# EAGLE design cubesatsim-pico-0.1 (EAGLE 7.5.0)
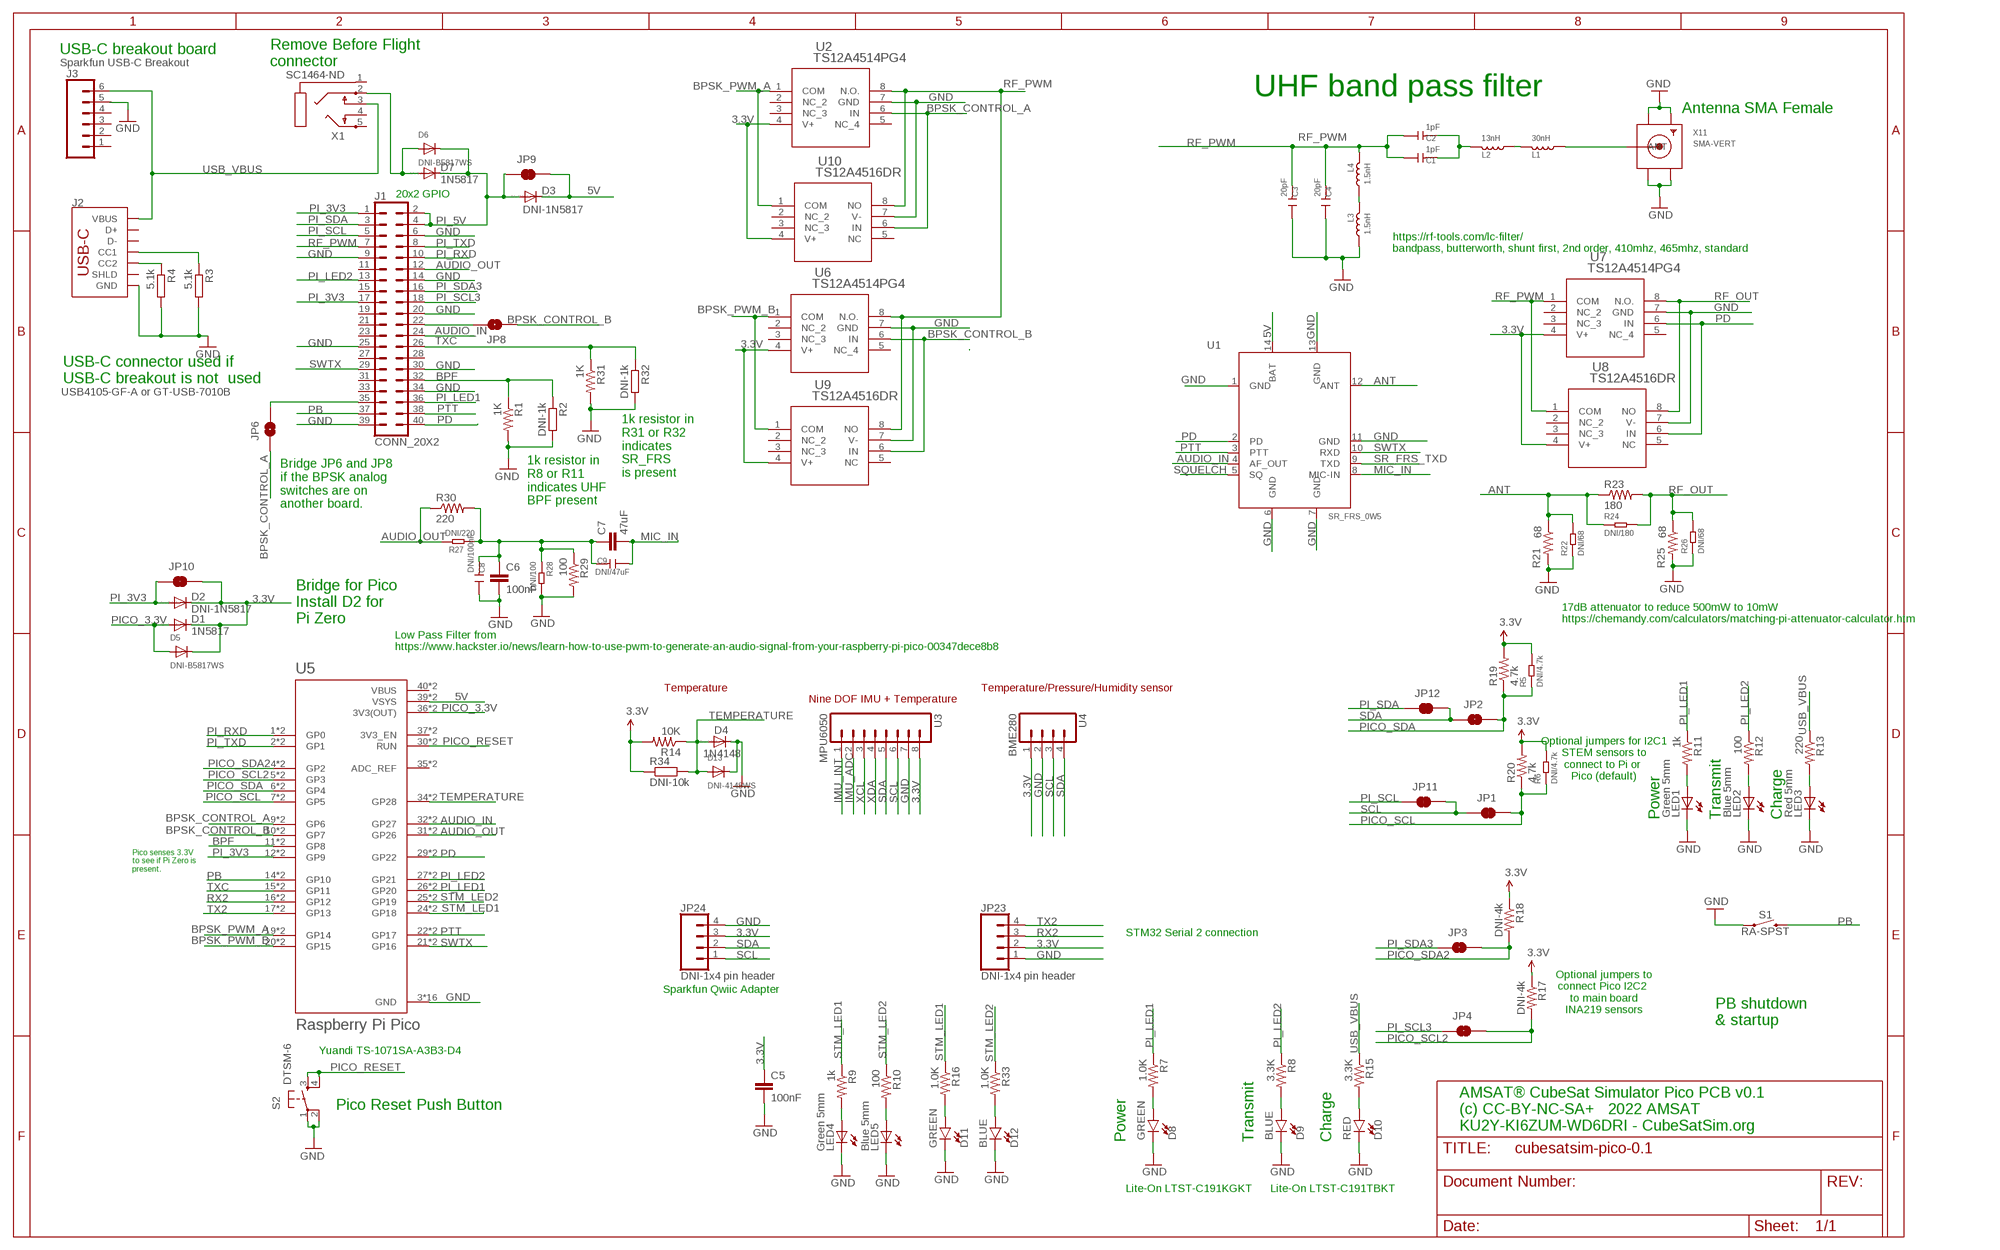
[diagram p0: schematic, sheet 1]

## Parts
C1  1pF  CERAMIC-10PF-50V-5%-NPO(0603)  [C0603]
C2  1pF  CERAMIC-10PF-50V-5%-NPO(0603)  [C0603]
C3  20pF  CERAMIC-10PF-50V-5%-NPO(0603)  [C0603]
C4  20pF  CERAMIC-10PF-50V-5%-NPO(0603)  [C0603]
C5  100nF  CAPPTH  [CAP-PTH-SMALL]
C6  100nF  CAPPTH  [CAP-PTH-SMALL]
C7  47uF  CAPPTH  [CAP-PTH-SMALL]
C8  DNI/100nF  CERAMIC-10PF-50V-5%-NPO(0603)  [C0603]
C9  DNI/47uF  CERAMIC-10PF-50V-5%-NPO(0603)  [C0603]
D1  1N5817  DIODE-D-2.5  [D-2.5]
D2  DNI-1N5817  DIODE-D-2.5  [D-2.5]
D3  DNI-1N5817  DIODE-D-2.5  [D-2.5]
D4  1N4148  DIODE-D-2.5  [D-2.5]
D5  DNI-B5817WS  DIODESOD-323F  [SOD-323F]
D6  DNI-B5817WS  DIODESOD-323F  [SOD-323F]
D7  1N5817  DIODE-D-2.5  [D-2.5]
D8  GREEN  LED-GREEN0603  [LED-0603]
D9  BLUE  LED-BLUE0603  [LED-0603]
D10  RED  LED-BLUE0603  [LED-0603]
D11  GREEN  LED-GREEN0603  [LED-0603]
D12  BLUE  LED-GREEN0603  [LED-0603]
D13  DNI-4148WS  DIODESOD-323F  [SOD-323F]
J1  CONN_20X2  [2X20]
J2  USB4105-GF-A or GT-USB-7010B  USB_C_2-LAYER_PADS  [USB-C-16P-2LAYER-PADS]
J3  Sparkfun USB-C Breakout  CONN_06NO_SILK_FEMALE_PTH  [1X06_NO_SILK]
JP1  JUMPER-SMT_2_NC_TRACE_SILK  [SMT-JUMPER_2_NC_TRACE_SILK]
JP2  JUMPER-SMT_2_NC_TRACE_SILK  [SMT-JUMPER_2_NC_TRACE_SILK]
JP3  JUMPER-SMT_2_NC_TRACE_SILK  [SMT-JUMPER_2_NC_TRACE_SILK]
JP4  JUMPER-SMT_2_NC_TRACE_SILK  [SMT-JUMPER_2_NC_TRACE_SILK]
JP6  JUMPER-SMT_2_NO_SILK  [SMT-JUMPER_2_NO_SILK]
JP8  JUMPER-SMT_2_NO_SILK  [SMT-JUMPER_2_NO_SILK]
JP9  JUMPER-SMT_2_NC_TRACE_SILK  [SMT-JUMPER_2_NC_TRACE_SILK]
JP10  JUMPER-SMT_2_NC_TRACE_SILK  [SMT-JUMPER_2_NC_TRACE_SILK]
JP11  JUMPER-SMT_2_NC_TRACE_SILK  [SMT-JUMPER_2_NC_TRACE_SILK]
JP12  JUMPER-SMT_2_NC_TRACE_SILK  [SMT-JUMPER_2_NC_TRACE_SILK]
JP23  DNI-1x4 pin header  CONN_041X04_NO_SILK  [1X04_NO_SILK]
JP24  DNI-1x4 pin header  CONN_041X04_NO_SILK  [1X04_NO_SILK]
L1  30nH  SMD-FERRITE-CHIP-120-OHM-500MA(0603)  [L0603]
L2  13nH  SMD-FERRITE-CHIP-120-OHM-500MA(0603)  [L0603]
L3  1.5nH  SMD-FERRITE-CHIP-120-OHM-500MA(0603)  [L0603]
L4  1.5nH  SMD-FERRITE-CHIP-120-OHM-500MA(0603)  [L0603]
LED1  Green 5mm  LED3MM  [LED3MM]
LED2  Blue 5mm  LED3MM  [LED3MM]
LED3  Red 5mm  LED3MM  [LED3MM]
LED4  Green 5mm  LED3MM  [LED3MM]
LED5  Blue 5mm  LED3MM  [LED3MM]
R1  1K  RESISTORPTH-1/4W-VERT-KIT  [AXIAL-0.1EZ]
R2  DNI-1k  R-EU_R0603  [R0603]
R3  5.1k  R-EU_R0603  [R0603]
R4  5.1k  R-EU_R0603  [R0603]
R5  DNI/4.7k  SMD-RES-1.2K-1%-1/10W(0603)  [R0603]
R6  DNI/4.7k  SMD-RES-1.2K-1%-1/10W(0603)  [R0603]
R7  1.0K  RESISTOR0603  [0603-RES]
R8  3.3K  RESISTOR0603-RES  [0603-RES]
R9  1k  RESISTORPTH-1/4W-VERT  [AXIAL-0.1]
R10  100  RESISTORPTH-1/4W-VERT  [AXIAL-0.1]
R11  1k  RESISTORPTH-1/4W-VERT-KIT  [AXIAL-0.1EZ]
R12  100  RESISTORPTH-1/4W-VERT-KIT  [AXIAL-0.1EZ]
R13  220  RESISTORPTH-1/4W-VERT-KIT  [AXIAL-0.1EZ]
R14  10K  RESISTORPTH-1/4W-VERT  [AXIAL-0.1]
R15  3.3K  RESISTOR0603-RES  [0603-RES]
R16  1.0K  RESISTOR0603  [0603-RES]
R17  DNI-4k  RESISTORPTH-1/4W-VERT  [AXIAL-0.1]
R18  DNI-4k  RESISTORPTH-1/4W-VERT  [AXIAL-0.1]
R19  4.7k  RESISTORPTH-1/4W-VERT  [AXIAL-0.1]
R20  4.7k  RESISTORPTH-1/4W-VERT  [AXIAL-0.1]
R21  68  RESISTORPTH-1/4W-VERT-KIT  [AXIAL-0.1EZ]
R22  DNI/68  SMD-RES-1.2K-1%-1/10W(0603)  [R0603]
R23  180  RESISTORPTH-1/4W-VERT-KIT  [AXIAL-0.1EZ]
R24  DNI/180  SMD-RES-1.2K-1%-1/10W(0603)  [R0603]
R25  68  RESISTORPTH-1/4W-VERT-KIT  [AXIAL-0.1EZ]
R26  DNI/68  SMD-RES-1.2K-1%-1/10W(0603)  [R0603]
R27  DNI/220  SMD-RES-1.2K-1%-1/10W(0603)  [R0603]
R28  DNI/100  SMD-RES-1.2K-1%-1/10W(0603)  [R0603]
R29  100  RESISTORPTH-1/4W-VERT-KIT  [AXIAL-0.1EZ]
R30  220  RESISTORPTH-1/4W-VERT-KIT  [AXIAL-0.1EZ]
R31  1K  RESISTORPTH-1/4W-VERT-KIT  [AXIAL-0.1EZ]
R32  DNI-1k  R-EU_R0603  [R0603]
R33  1.0K  RESISTOR0603  [0603-RES]
R34  DNI-10k  R-EU_R0603  [R0603]
S1  RA-SPST  [RA-SPST]
S2  DTSM-6  [DTSM-6]
U1  SR_FRS_0W5  [SR_FRS_0W5]
U2  TS12A4514PG4  TS12A4515PG4  [P8_TEX]
U3  MPU6050  M08NO_SILK_FEMALE_PTH  [1X08_NO_SILK]
U4  BME280  M04NO_SILK_ALL_ROUND  [1X04_NO_SILK_ALL_ROUND]
U5  Raspberry Pi Pico  RASPBERRY_PICO-NO_DEBUG  [PICO-PKG-NO_DEBUG]
U6  TS12A4514PG4  TS12A4515PG4  [P8_TEX]
U7  TS12A4514PG4  TS12A4515PG4  [P8_TEX]
U8  TS12A4516DR  [D8]
U9  TS12A4516DR  [D8]
U10  TS12A4516DR  [D8]
X1  SC1464-ND  PG203J  [PG203J]
X11  SMA-VERT  [SMA-VERT]

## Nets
3.3V: C5.1 D1.C D2.C D5.C JP10.2 JP23.2 JP24.3 R5.2 R6.2 R14.P$2 R17.P$1 R18.P$1 R19.P$2 R20.P$2 R34.1 U2.4(V+) U3.8 U4.1 U6.4(V+) U7.4(V+) U8.4(V+) U9.4(V+) U10.4(V+)
5V: D3.C JP9.2 U1.14(BAT) U5.39(VSYS) U5.P$39(VSYS)
ANT: R21.P$1 R22.2 R23.P$1 R24.1 U1.12(ANT)
AUDIO_IN: J1.24 U1.4(AF_OUT) U5.32(GP27) U5.P$32(GP27)
AUDIO_OUT: J1.12 R27.2 R30.P$1 U5.31(GP26) U5.P$31(GP26)
BPF: J1.32 R1.P$1 R2.1 U5.11(GP8) U5.P$11(GP8)
BPSK_CONTROL_A: JP6.1 U2.6(IN) U5.9(GP6) U5.P$9(GP6) U10.6(IN)
BPSK_CONTROL_B: JP8.1 U5.10(GP7) U5.P$10(GP7) U6.6(IN) U9.6(IN)
BPSK_PWM_A: U2.1(COM) U5.19(GP14) U5.P$19(GP14) U10.1(COM)
BPSK_PWM_B: U5.20(GP15) U5.P$20(GP15) U6.1(COM) U9.1(COM)
GND: C3.1 C4.1 C5.2 C6.2 C8.1 D4.C D8.C D9.C D10.C D11.C D12.C D13.C J1.6 J1.9 J1.14 J1.20 J1.25 J1.30 J1.34 J1.39 J2.GND J2.GND2(GND) J3.5 JP23.1 JP24.4 L3.2 LED1.K(C) LED2.K(C) LED3.K(C) LED4.K(C) LED5.K(C) R1.P$2 R2.2 R3.2 R4.2 R21.P$2 R22.1 R25.P$2 R26.1 R28.2 R29.P$2 R31.P$2 R32.2 S1.1 S2.1 S2.2 U1.1(GND) U1.6(GND) U1.7(GND) U1.11(GND) U1.13(GND) U2.7(GND) U3.7 U4.2 U5.3(GND) U5.8(GND) U5.13(GND) U5.18(GND) U5.23(GND) U5.28(GND) U5.33(GND) U5.38(GND) U5.P$3(GND) U5.P$8(GND) U5.P$13(GND) U5.P$18(GND) U5.P$23(GND) U5.P$28(GND) U5.P$33(GND) U5.P$38(GND) U6.7(GND) U7.7(GND) U8.7(V-) U9.7(V-) U10.7(V-) X11.GND1 X11.GND2 X11.GND3 X11.GND4
IMU_ADC: U3.2
IMU_INT: U3.1
MIC_IN: C7.2 C9.1 U1.8(MIC-IN)
N$3: LED4.A R9.P$2
N$4: LED5.A R10.P$2
N$5: C6.1 C7.1 C8.2 C9.2 R27.1 R28.1 R29.P$1 R30.P$2
N$6: LED1.A R11.P$2
N$8: L1.2 X11.ANTENNA(ANT)
N$9: LED2.A R12.P$2
N$10: C1.2 C2.2 L2.1
N$11: LED3.A R13.P$2
N$22: J1.35 JP6.2
N$23: J2.B5(CC2) R4.1
N$24: J2.A5(CC1) R3.1
N$25: J1.22 JP8.2
N$27: D8.A R7.2
N$28: L3.1 L4.2
N$29: D9.A R8.2
N$30: D10.A R15.2
N$31: D11.A R16.2
N$32: D12.A R33.2
N$50: L1.1 L2.2
PB: J1.37 S1.2 U5.14(GP10) U5.P$14(GP10)
PD: J1.40 U1.2(PD) U5.29(GP22) U5.P$29(GP22) U7.6(IN) U8.6(IN)
PI_3V3: D2.A J1.1 J1.17 JP10.1 U5.12(GP9) U5.P$12(GP9)
PI_5V: D3.A D6.C D7.C J1.2 J1.4 JP9.1
PI_LED1: J1.36 R7.1 R11.P$1 U5.26(GP20) U5.P$26(GP20)
PI_LED2: J1.13 R8.1 R12.P$1 U5.27(GP21) U5.P$27(GP21)
PI_RXD: J1.10 U5.1(GP0) U5.P$1(GP0)
PI_SCL: J1.5 JP11.1
PI_SCL3: J1.18 JP4.1
PI_SDA: J1.3 JP12.1
PI_SDA3: J1.16 JP3.1
PI_TXD: J1.8 U5.2(GP1) U5.P$2(GP1)
PICO_3.3V: D1.A D5.A U5.36(3V3(OUT)) U5.P$36(3V3(OUT))
PICO_3.3V1: D6.A D7.A X1.2
PICO_RESET: S2.3 S2.4 U5.30(RUN) U5.P$30(RUN)
PICO_SCL: JP1.2 R6.1 R20.P$1 U5.7(GP5) U5.P$7(GP5)
PICO_SCL2: JP4.2 R17.P$2 U5.5(GP3) U5.P$5(GP3)
PICO_SDA: JP2.2 R5.1 R19.P$1 U5.6(GP4) U5.P$6(GP4)
PICO_SDA2: JP3.2 R18.P$2 U5.4(GP2) U5.P$4(GP2)
PTT: J1.38 U1.3(PTT) U5.22(GP17) U5.P$22(GP17)
RF_OUT: R23.P$2 R24.2 R25.P$1 R26.2 U7.8(N.O.) U8.8(NO)
RF_PWM: C1.1 C2.1 C3.2 C4.2 J1.7 L4.1 U2.8(N.O.) U6.8(N.O.) U7.1(COM) U8.1(COM) U9.8(NO) U10.8(NO)
RX2: JP23.3 U5.16(GP12) U5.P$16(GP12)
SCL: JP1.1 JP11.2 JP24.1 U3.6 U4.3
SDA: JP2.1 JP12.2 JP24.2 U3.5 U4.4
SQUELCH: U1.5(SQ)
SR_FRS_TXD: U1.9(TXD)
STM_LED1: R9.P$1 R16.1 U5.24(GP18) U5.P$24(GP18)
STM_LED2: R10.P$1 R33.1 U5.25(GP19) U5.P$25(GP19)
SWTX: J1.29 U1.10(RXD) U5.21(GP16) U5.P$21(GP16)
TEMPERATURE: D4.A D13.A R14.P$1 R34.2 U5.34(GP28) U5.P$34(GP28)
TX2: JP23.4 U5.17(GP13) U5.P$17(GP13)
TXC: J1.26 R31.P$1 R32.1 U5.15(GP11) U5.P$15(GP11)
USB_VBUS: J2.VBUS1(VBUS) J2.VBUS2(VBUS) J3.6 R13.P$1 R15.1 X1.3
XCL: U3.3
XDA: U3.4
Unconnected: J1.11 J1.15 J1.19 J1.21 J1.23 J1.27 J1.28 J1.31 J1.33 J2.A6(D+) J2.A7(D-) J2.B6(D+) J2.B7(D-) J2.SHLD1(SHLD) J2.SHLD2(SHLD) J2.SHLD3(SHLD) J2.SHLD4(SHLD) J3.1 J3.2 J3.3 J3.4 U2.2(NC_2) U2.3(NC_3) U2.5(NC_4) U5.35(ADC_REF) U5.37(3V3_EN) U5.P$35(ADC_REF) U5.P$37(3V3_EN) U6.2(NC_2) U6.3(NC_3) U6.5(NC_4) U7.2(NC_2) U7.3(NC_3) U7.5(NC_4) U8.2(NC_2) U8.3(NC_3) U8.5(NC) U9.2(NC_2) U9.3(NC_3) U9.5(NC) U10.2(NC_2) U10.3(NC_3) U10.5(NC) X1.1 X1.4 X1.5

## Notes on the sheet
- USB-C breakout board
- Remove Before Flight
  connector
- UHF band pass filter
- Antenna SMA Female
- 20x2 GPIO
- https://rf-tools.com/lc-filter/
  bandpass, butterworth, shunt first, 2nd order, 410mhz, 465mhz, standard
- USB-C connector used if 
  USB-C breakout is not  used
- 1k resistor in 
  R31 or R32
  indicates 
  SR_FRS 
  is present
- 1k resistor in 
  R8 or R11
  indicates UHF 
  BPF present
- Bridge JP6 and JP8
  if the BPSK analog
  switches are on
  another board.
- 17dB attenuator to reduce 500mW to 10mW
  https://chemandy.com/calculators/matching-pi-attenuator-calculator.htm
- Bridge for Pico
  Install D2 for
  Pi Zero
- Low Pass Filter from
  https://www.hackster.io/news/learn-how-to-use-pwm-to-generate-an-audio-signal-from-your-raspberry-pi-pico-00347dece8b8
- Temperature | Temperature/Pressure/Humidity sensor
- Nine DOF IMU + Temperature
- Optional jumpers for I2C1
  STEM sensors to
  connect to Pi or 
  Pico (default)
- Power | Transmit | Charge
- Pico senses 3.3V 
  to see if Pi Zero is
  present.
- STM32 Serial 2 connection
- Optional jumpers to
  connect Pico I2C2 
  to main board
  INA219 sensors
- Sparkfun Qwiic Adapter
- PB shutdown
  & startup
- Yuandi TS-1071SA-A3B3-D4
- Pico Reset Push Button
- AMSAT® CubeSat Simulator Pico PCB v0.1
  (c) CC-BY-NC-SA+   2022 AMSAT
  KU2Y-KI6ZUM-WD6DRI - CubeSatSim.org
- Power | Transmit | Charge
- Lite-On LTST-C191KGKT | Lite-On LTST-C191TBKT

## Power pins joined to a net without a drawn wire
VBUS: U5.40(VBUS) U5.P$40(VBUS)

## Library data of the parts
C1-C4 C8 C9 = Seeed-OPL-Capacitor:CERAMIC-10PF-50V-5%-NPO(0603): 302010097; VALUE: 10pf
C5-C7 = SparkFun-Capacitors:CAP: Capacitor
D1-D4 D7 = diode:DIODE-: DIODE
D5 D6 D13 = adafruit:DIODE: Diode
D8 D11 = SparkFun-LED:LED-GREEN: Green SMD LED; PROD_ID: DIO-00821
D9 = SparkFun-LED:LED-BLUE: Blue SMD LED; PROD_ID: DIO-08575
D10 = SparkFun-LED:LED-BLUE: Blue SMD LED; PROD_ID: DIO-08575; VALUE: BLUE
D12 = SparkFun-LED:LED-GREEN: Green SMD LED; PROD_ID: DIO-00821; VALUE: GREEN
J1 = SparkFun-Connectors-AJ2:CONN_20X2: Multi connection point. Often used as Generic Header-pin footprint for 0.1 inch spaced/style header connections On any of the 0.1 inch spaced packages, you can populate with these: Break Away Headers - Straight (PRT-00116) Break Away Male Headers - Right Angle (PRT-00553) Female Headers (PRT-00115)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
J2 = SparkFun-Connectors:USB_C: USB Type C 16Pin Connector Super Speed pins not available on the 16-pin purely SMD connector so this part is best for USB 2.0 implementations. D1 and D2 are tied together enabling D+/- no matter which way the cable is plugged into the connector. The two channel configuration pins (CC1/2) are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; PROD_ID: CONN-14122
J3 = SparkFun-Connectors-AJ-3:CONN_06: Multi connection point. Often used as Generic Header-pin footprint for 0.1 inch spaced/style header connections On any of the 0.1 inch spaced packages, you can populate with these: Break Away Headers - Straight (PRT-00116) Break Away Male Headers - Right Angle (PRT-00553) Female Headers (PRT-00115)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; PROD_ID: CONN-08437
JP1-JP4 JP9-JP12 = SparkFun-Jumpers:JUMPER-SMT_2_NC_TRACE: Normally closed trace jumper
JP6 JP8 = SparkFun-Jumpers:JUMPER-SMT_2_NO: Normally open jumper
JP23 JP24 = SparkFun-Connectors:CONN_04: Multi connection point. Often used as Generic Header-pin footprint for 0.1 inch spaced/style header connections On any of the 0.1 inch spaced packages, you can populate with these: Break Away Headers - Straight (PRT-00116) Break Away Male Headers - Right Angle (PRT-00553) Female Headers (PRT-00115)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; PROD_ID: CONN-09696
L1-L4 = Seeed-OPL-Inductor:SMD-FERRITE-CHIP-120-OHM-500MA(0603): 303030001; MPN: BLM18AG121SN1D; VALUE: 120
LED1-LED5 = adafruit:LED: LED
R1 R7-R21 R23 R25 R29-R31 R33 = SparkFun-Resistors:RESISTOR: Resistor
R2-R4 R32 R34 = resistor:R-EU_: RESISTOR, European symbol
R5 R6 R22 R24 R26-R28 = Seeed-OPL-Resistor:SMD-RES-1.2K-1%-1/10W(0603): 301010206; MPN: RC0603FR-071K2L; VALUE: 1.2K
S1 = zumradio:RA-SPST
S2 = switch-tact-aj:DTSM-6
U1 = SR_FRS_0W5:SR_FRS_0W5
U2 U6 U7 = TS12A4514:TS12A4515PG4; COPYRIGHT: Copyright (C) 2022 Ultra Librarian. All rights reserved.; MANUFACTURER_PART_NUMBER: TS12A4515PG4; MFR_NAME: Texas Instruments
U3 = SparkFun-Connectors:M08: Header 8 Standard 8-pin 0.1" header. Use with straight break away headers (SKU : PRT-00116), right angle break away headers (PRT-00553), swiss pins (PRT-00743), machine pins (PRT-00117), and female headers (PRT-00115).; PROD_ID: CONN-08438
U4 = SparkFun-Connectors:M04: Header 4 Standard 4-pin 0.1" header. Use with straight break away headers (SKU : PRT-00116), right angle break away headers (PRT-00553), swiss pins (PRT-00743), machine pins (PRT-00117), and female headers (PRT-00115). Molex polarized connector foot print use with SKU : PRT-08231 with associated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
U5 = RpiPico:RASPBERRY_PICO-NO_DEBUG
U8-U10 = TS12A4514-soic:TS12A4516DR; COPYRIGHT: Copyright (C) 2022 Ultra Librarian. All rights reserved.; DIGI-KEY_PART_NUMBER_1: 296-21911-1-ND; DIGI-KEY_PART_NUMBER_2: 296-21911-2-ND; DIGI-KEY_PART_NUMBER_3: 296-21911-6-ND; DIGI-KEY_PART_NUMBER_4: 2156-TS12A4516DR-ND; MANUFACTURER_PART_NUMBER: TS12A4516DR; MFR_NAME: Texas Instruments
X1 = con-hirschmann:PG203J: MIC/HEADPHONE JACK KS-S stereo microphone/headphone jack PG203JN (Schukat); OC_FARNELL: unknown; OC_NEWARK: unknown
X11 = zum_radio:SMA-VERT

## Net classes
1 RF: clearance 0.381 mm

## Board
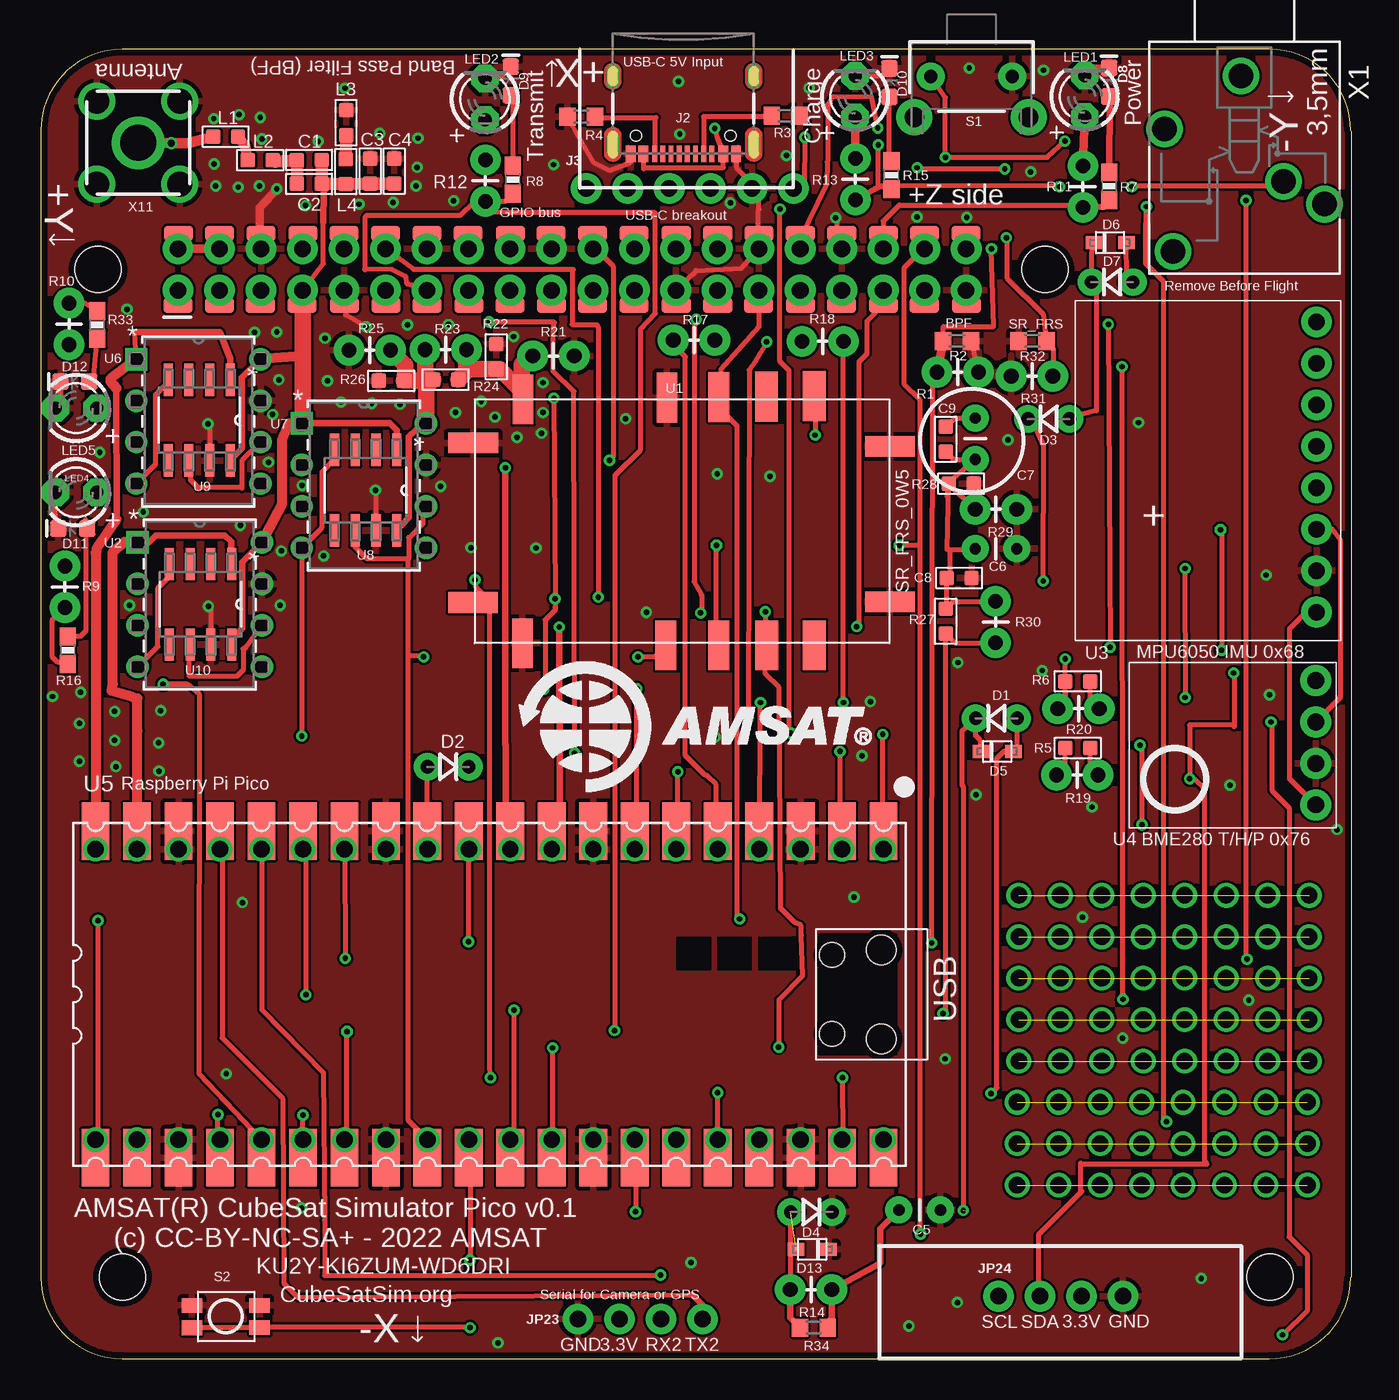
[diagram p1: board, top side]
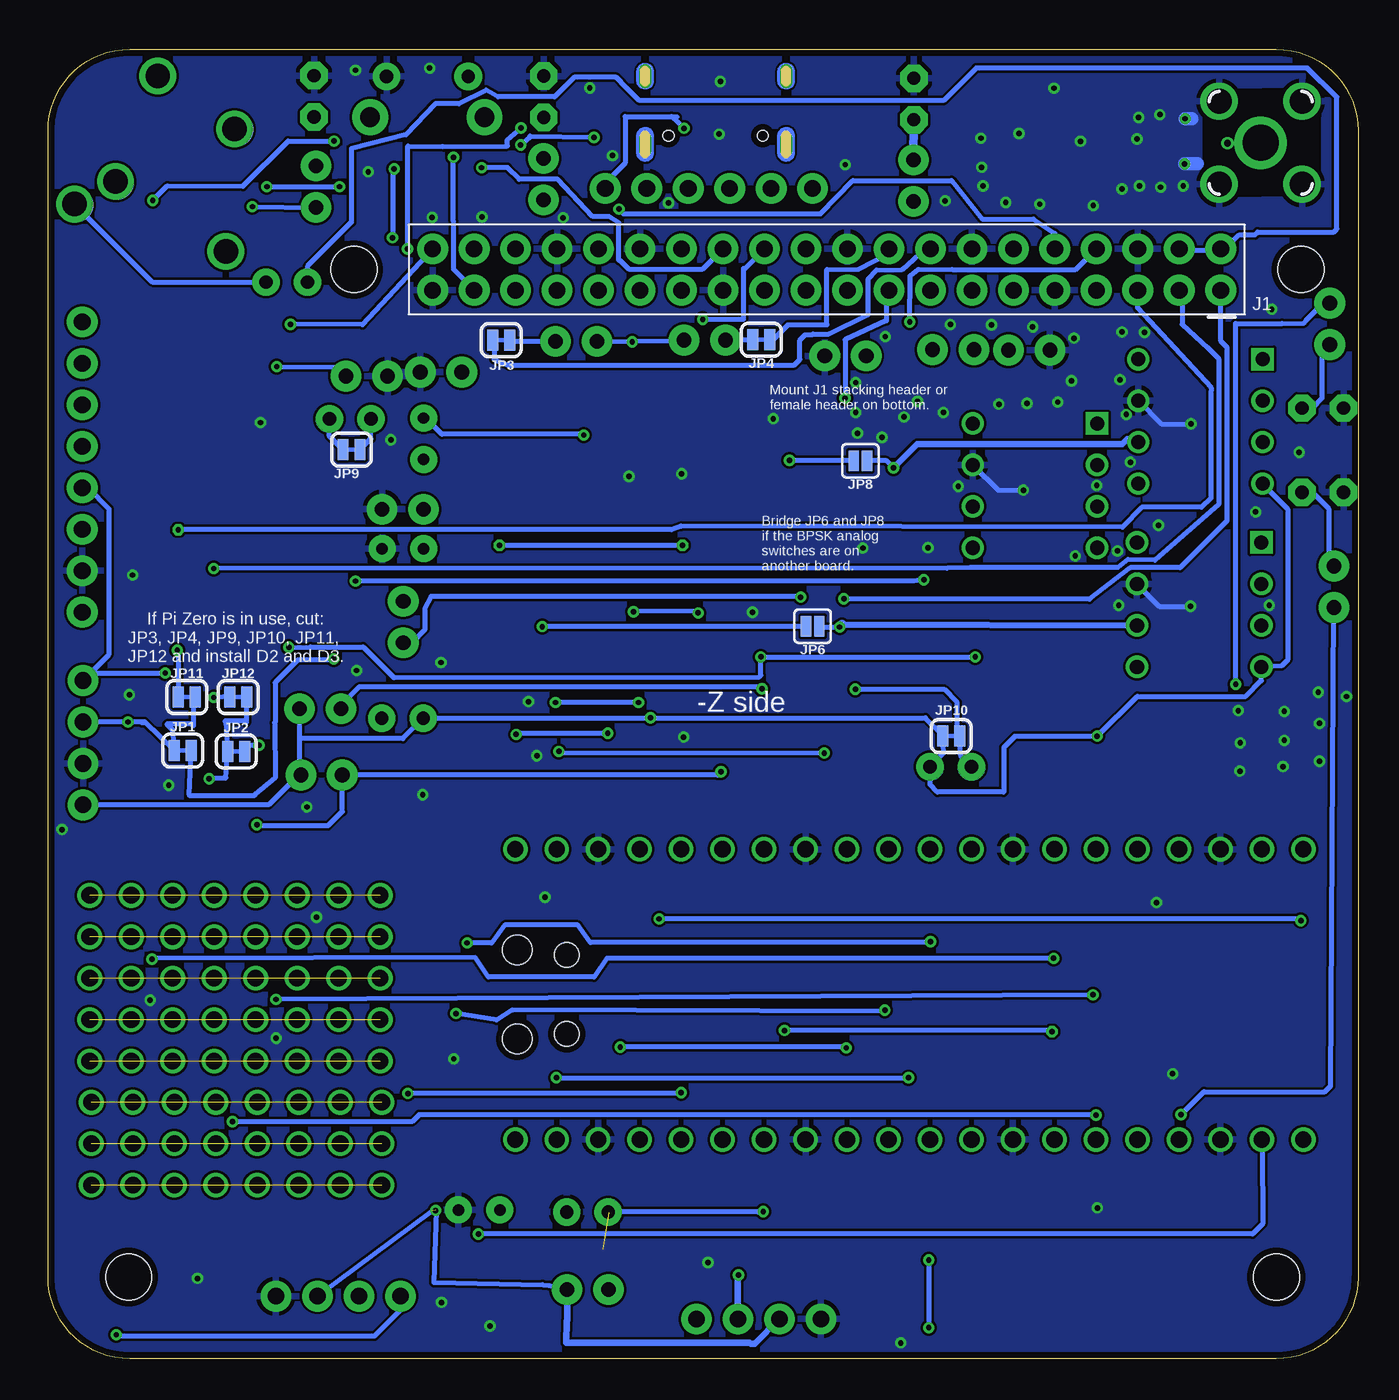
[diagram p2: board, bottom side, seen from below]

Size 80.24 x 80.23 mm. Coordinates in mm from the lower left corner, seen from the top.
Outline: 80.23,5 arc-90 75.23,0 5,0 arc-90 0,5 0,75.23 arc-90 5,80.23 75.23,80.23 arc-90 80.23,75.23
Outline: 80.24,75.2 80.24,4.98
Copper layers (1*16): Top 0.0356mm / dielectric 1.5011mm / Bottom 0.0356mm
Design rules "LaenPCBOrder *": minimum track width 6mil, minimum drill 13mil, track to track 6mil, track to pad 6mil, pad to pad 6mil, via to via 6mil, smd to smd 6mil, copper to edge 15mil, drill to drill 6mil, minimum pad ring 7mil, minimum via ring 7mil, stop-mask expansion 3mil, vias tented up to drill 25mil, thermal gap 10mil
Holes 2.8 mm at 3.5,66.73 61.5,66.73 75.28,5 5,5

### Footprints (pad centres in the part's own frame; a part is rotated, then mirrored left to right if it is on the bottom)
C0603 = smd 0.889 x 0.889: 1 0,0.762; 2 0,-0.762
CAP-PTH-SMALL = drill 0.7 pad 1.651: 1 0,0; 2 2.54,0
D-2.5 = drill 0.813 pad 1.676: A 1.27,0; C -1.27,0 | smd 1.676 x 1.676 bottom: P$1 -1.27,0; P$2 1.27,0
SOD-323F = smd 1 x 0.8: A -1,0; C 1,0
LED-0603 = smd 1 x 1: A -0.877,0; C 0.877,0
2X20 = drill 1.016 pad 1.88: 1 -24.13,-1.27; 2 -24.13,1.27; 3 -21.59,-1.27; 4 -21.59,1.27; 5 -19.05,-1.27; 6 -19.05,1.27; 7 -16.51,-1.27; 8 -16.51,1.27; 9 -13.97,-1.27; 10 -13.97,1.27; 11 -11.43,-1.27; 12 -11.43,1.27; 13 -8.89,-1.27; 14 -8.89,1.27; 15 -6.35,-1.27; 16 -6.35,1.27; 17 -3.81,-1.27; 18 -3.81,1.27; 19 -1.27,-1.27; 20 -1.27,1.27; 21 1.27,-1.27; 22 1.27,1.27; 23 3.81,-1.27; 24 3.81,1.27; 25 6.35,-1.27; 26 6.35,1.27; 27 8.89,-1.27; 28 8.89,1.27; 29 11.43,-1.27; 30 11.43,1.27; 31 13.97,-1.27; 32 13.97,1.27; 33 16.51,-1.27; 34 16.51,1.27; 35 19.05,-1.27; 36 19.05,1.27; 37 21.59,-1.27; 38 21.59,1.27; 39 24.13,-1.27; 40 24.13,1.27 | smd 1.778 x 0.914: P$1 -19.05,2.21; P$4 -16.485,2.21; P$10 -21.59,2.21; P$11 -24.117,2.223; P$12 -13.97,2.21; P$13 -11.43,2.21; P$14 -8.89,2.21; P$16 -6.375,2.21; P$17 -3.785,2.21; P$20 -1.295,2.21; P$21 1.245,2.21; P$22 3.785,2.21; P$23 6.375,2.21; P$27 8.915,2.21; P$28 11.43,2.21; P$29 13.97,2.21; P$30 16.51,2.21; P$31 19.075,2.21; P$32 21.59,2.21; P$33 24.13,2.21; P$41 -19.101,-2.21; P$44 -16.535,-2.21; P$50 -21.59,-2.21; P$51 -24.13,-2.21; P$52 -13.945,-2.21; P$53 -11.405,-2.21; P$54 -8.89,-2.21; P$56 -6.325,-2.21; P$57 -3.81,-2.21; P$60 -1.27,-2.21; P$61 1.245,-2.21; P$62 3.785,-2.21; P$63 6.375,-2.21; P$67 8.915,-2.21; P$68 11.405,-2.21; P$69 13.995,-2.21; P$70 16.485,-2.21; P$71 19.075,-2.21; P$72 21.565,-2.21; P$73 24.155,-2.21
USB-C-16P-2LAYER-PADS = smd 0.3 x 1: A5 -1.25,-0.34; A6 -0.25,-0.34; A7 0.25,-0.34; A8 1.25,-0.34; B5 1.75,-0.34; B6 0.75,-0.34; B7 -0.75,-0.34; B8 -1.75,-0.34 | smd 0.6 x 1: GND -3.225,-0.34; GND2 3.225,-0.34; VBUS1 -2.45,-0.34; VBUS2 2.45,-0.34 | drill 0.4 pad 0.6 long: SHLD1 -4.318,-0.915; SHLD2 4.318,-0.915; SHLD3 -4.318,-5.095; SHLD4 4.318,-5.095 | hole 0.65: -2.89,-1.445; 2.89,-1.445
1X06_NO_SILK = drill 1.016 pad 1.88: 1 0,0; 2 2.54,0; 3 5.08,0; 4 7.62,0; 5 10.16,0; 6 12.7,0 | smd 1.905 x 1.905 bottom: P$2 2.54,0; P$7 0,0; P$8 5.08,0; P$9 7.62,0; P$22 10.16,0; P$23 12.7,0
SMT-JUMPER_2_NC_TRACE_SILK = smd 0.66 x 1.27: 1 -0.521,0; 2 0.521,0
SMT-JUMPER_2_NO_SILK = smd 0.635 x 1.27: 1 -0.406,0; 2 0.406,0
1X04_NO_SILK = drill 1.016 pad 1.88: 1 0,0; 2 2.54,0; 3 5.08,0; 4 7.62,0
L0603 = smd 0.889 x 0.889: 1 -0.762,0; 2 0.762,0
LED3MM = drill 0.813 pad 1.676 octagon: A -1.27,0; K 1.27,0
AXIAL-0.1EZ = drill 0.9 pad 1.88: P$1 0,0; P$2 2.54,0
R0603 = smd 1 x 1.1: 1 -0.85,0; 2 0.85,0
R0603' = smd 0.889 x 0.889: 1 0,0.762; 2 0,-0.762
0603-RES = smd 1.1 x 1: 1 -0.85,0; 2 0.85,0
AXIAL-0.1 = drill 0.9 pad 1.88: P$1 0,0; P$2 2.54,0
RA-SPST = drill 0.8 pad 1.7: 1 -2.5,0; 2 2.5,0 | drill 1.2 pad 2.2: ANCHOR1 -3.5,2.5; ANCHOR2 3.5,2.5
DTSM-6 = smd 1.25 x 0.9: 1 -2.125,0.6; 2 2.025,0.6; 3 -2.125,-0.76; 4 2.025,-0.75
SR_FRS_0W5 = smd 3.048 x 1.27: 1 7.06,-9.694; 2 7.187,-0.926; 3 7.187,2.33; 10 -8.014,2.329; 11 -7.986,-0.846; 12 -7.876,-9.664 | smd 3.048 x 1.397: 4 7.187,5.256; 5 7.187,8.182; 9 -8.042,5.25 | smd 1.27 x 3.048: 6 4.52,12.81; 7 -5.005,12.815; 13 -5.209,-12.717; 14 4.57,-12.722 | smd 3.048 x 1.422: 8 -8.07,8.171
P8_TEX = drill 0.864 pad 1.372 square: 1 0,0 | drill 0.864 pad 1.372: 2 0,-2.54; 3 0,-5.08; 4 0,-7.62; 5 7.62,-7.62; 6 7.62,-5.08; 7 7.62,-2.54; 8 7.62,0
1X08_NO_SILK = drill 1.016 pad 1.88: 1 0,0; 2 2.54,0; 3 5.08,0; 4 7.62,0; 5 10.16,0; 6 12.7,0; 7 15.24,0; 8 17.78,0
1X04_NO_SILK_ALL_ROUND = drill 1.016 pad 1.88: 1 0,0; 2 2.54,0; 3 5.08,0; 4 7.62,0
PICO-PKG-NO_DEBUG = drill 1: 1 -7.62,25.4; 2 -7.62,22.86; 3 -7.62,20.32; 4 -7.62,17.78; 5 -7.62,15.24; 6 -7.62,12.7; 7 -7.62,10.16; 8 -7.62,7.62; 9 -7.62,5.08; 10 -7.62,2.54; 11 -7.62,0; 12 -7.62,-2.54; 13 -7.62,-5.08; 14 -7.62,-7.62; 15 -7.62,-10.16; 16 -7.62,-12.7; 17 -7.62,-15.24; 18 -7.62,-17.78; 19 -7.62,-20.32; 20 -7.62,-22.86; 21 10.16,-22.86; 22 10.16,-20.32; 23 10.16,-17.78; 24 10.16,-15.24; 25 10.16,-12.7; 26 10.16,-10.16; 27 10.16,-7.62; 28 10.16,-5.08; 29 10.16,-2.54; 30 10.16,0; 31 10.16,2.54; 32 10.16,5.08; 33 10.16,7.62; 34 10.16,10.16; 35 10.16,12.7; 36 10.16,15.24; 37 10.16,17.78; 38 10.16,20.32; 39 10.16,22.86; 40 10.16,25.4 | smd 3.5 x 1.7: P$1 -8.73,25.4; P$2 -8.73,22.86; P$3 -8.73,20.32; P$4 -8.73,17.78; P$5 -8.73,15.24; P$6 -8.73,12.7; P$7 -8.73,10.16; P$8 -8.73,7.62; P$9 -8.73,5.08; P$10 -8.73,2.54; P$11 -8.73,0; P$12 -8.73,-2.54; P$13 -8.73,-5.08; P$14 -8.73,-7.62; P$15 -8.73,-10.16; P$16 -8.73,-12.7; P$17 -8.73,-15.24; P$18 -8.73,-17.78; P$19 -8.73,-20.32; P$20 -8.73,-22.86; P$21 11.27,-22.86; P$22 11.27,-20.32; P$23 11.27,-17.78; P$24 11.27,-15.24; P$25 11.27,-12.7; P$26 11.27,-10.16; P$27 11.27,-7.62; P$28 11.27,-5.08; P$29 11.27,-2.54; P$30 11.27,0; P$31 11.27,2.54; P$32 11.27,5.08; P$33 11.27,7.62; P$34 11.27,10.16; P$35 11.27,12.7; P$36 11.27,15.24; P$37 11.27,17.78; P$38 11.27,20.32; P$39 11.27,22.86; P$40 11.27,25.4 | hole 1.8: -1.455,25.27; 3.995,25.27 | hole 1.5: -1.155,22.24; 3.695,22.24
D8 = smd 1.981 x 0.559: 1 -2.464,1.905; 2 -2.464,0.635; 3 -2.464,-0.635; 4 -2.464,-1.905; 5 2.464,-1.905; 6 2.464,-0.635; 7 2.464,0.635; 8 2.464,1.905
PG203J = drill 1.499: 1 -5.004,-0.203; 2 2.845,4.902; 3 1.448,2.388; 4 5.74,-4.369; 5 -1.753,-4.902 | smd 2.159 x 2.159 bottom: P$1 -5.004,-0.178; P$2 -1.727,-5.004; P$3 1.524,2.337; P$4 2.896,4.801; P$5 5.715,-4.369
SMA-VERT = drill 2.2: ANTENNA 0,0 | drill 1.524: GND1 -2.54,2.54; GND2 2.54,2.54; GND3 -2.54,-2.54; GND4 2.54,-2.54

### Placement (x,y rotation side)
C1  16.43,73.44 270 top
C2  16.43,71.98 270 top
C3  20.17,72.75 0 top
C4  21.64,72.75 0 top
C5  52.55,9.11 0 top
C6  57.23,49.62 0 top
C7  57.23,55.09 90 top
C8  56.24,47.82 270 top
C9  55.42,56.33 0 top
D1  58.52,39.24 0 top
D2  24.94,36.26 180 top
D3  61.72,57.57 0 top
D4  47.19,8.98 180 top
D5  58.57,37.2 180 top
D6  65.48,68.37 180 top
D7  65.61,65.96 0 top
D8  65.43,78.2 90 top
D9  28.78,78.28 90 top
D10  51.97,78.17 90 top
D11  1.96,50.87 180 top
D12  2.08,59.86 180 top
D13  47.24,6.7 0 top
J1  32.54,66.73 0 top
J2  39.34,73.48 180 top
J3  33.4,71.7 0 top
JP1  71.98,37.25 0 bottom
JP2  68.71,37.2 0 bottom
JP3  52.48,62.4 0 bottom
JP4  36.55,62.43 180 bottom
JP6  33.4,44.87 180 bottom
JP8  30.48,55.01 180 bottom
JP9  61.65,55.7 0 bottom
JP10  24.92,38.14 180 bottom
JP11  71.73,40.53 0 bottom
JP12  68.58,40.53 0 bottom
JP23  32.89,2.43 0 top
JP24  58.65,3.83 0 top
L1  11.32,74.86 180 top
L2  13.44,73.42 180 top
L3  18.69,75.72 90 top
L4  18.67,72.73 90 top
LED1  63.93,77.34 90 top
LED2  27.2,77.17 90 top
LED3  49.87,77.31 90 top
LED4  2.16,53.08 180 top
LED5  2.16,58.24 180 top
R1  54.89,60.45 0 top
R2  56.11,62.35 0 top
R3  45.62,76.14 0 top
R4  33.1,76.09 180 top
R5  DNI/4.7k  [R0603']  63.5,37.41 90 top
R6  DNI/4.7k  [R0603']  63.5,41.5 90 top
R7  65.43,71.82 90 top
R8  28.91,72.23 90 top
R9  1.47,46.02 90 top
R10  1.73,64.66 270 top
R11  63.82,70.53 90 top
R12  27.23,70.9 90 top
R13  49.89,70.99 90 top
R14  45.9,4.23 0 top
R15  52.1,72.51 90 top
R16  1.65,43.4 90 top
R17  41.27,62.4 180 top
R18  46.61,62.32 0 top
R19  62.2,35.76 0 top
R20  62.28,39.82 0 top
R21  30.12,61.44 0 top
R22  DNI/68  [R0603']  27.89,61.38 0 top
R23  26.06,61.82 180 top
R24  DNI/180  [R0603']  24.79,59.99 270 top
R25  21.41,61.79 180 top
R26  DNI/68  [R0603']  21.46,59.91 90 top
R27  DNI/220  [R0603']  55.42,45.18 0 top
R28  DNI/100  [R0603']  56.36,53.61 90 top
R29  57.23,52.04 0 top
R30  58.47,43.86 90 top
R31  61.98,60.19 180 top
R32  60.73,62.35 180 top
R33  3.45,63.34 270 top
R34  47.35,1.9 180 top
S1  57,78.56 180 top
S2  11.38,2.66 0 top
U1  39.19,50.89 270 top
U2  5.92,50.01 0 top
U3  78.13,63.52 270 top
U4  78.08,33.93 90 top
U5  26.21,23.59 270 top
U6  5.84,61.23 0 top
U7  15.98,57.3 0 top
U8  19.89,53.21 270 top
U9  9.7,57.5 270 top
U10  9.78,46.22 270 top
X1  73.71,73.58 270 top
X11  5.97,74.49 180 bottom

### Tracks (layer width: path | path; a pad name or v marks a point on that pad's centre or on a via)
3.3V  (via drill 0.33)  (1 unrouted)
  Top 0.305: R6.2 64.24,41.29 64.24,40.1 64.52,39.82 R20.P$2 | R19.P$2 64.26,36.24 R5.2 | D5.C 57.56,36.94 57.56,37.86 57.25,38.17 D1.C 56.41,38.45 56.41,35.15 56.49,35.07 v56.49,9.09 | v44.45,62.3 44.48,62.3 43.79,61.13 43.38,60.57 v43.33,39.26 | U4.1 76.48,35.53 76.48,44.72 77.5,45.74 U3.8 | U8.4 17.98,55.09 17.22,54.32 17.22,50.92 U7.4 v15.98,38.14 | U6.4 7.04,54.81 7.04,59.07 7.8,59.84 U9.4 | U2.4 7.16,43.63 7.16,47.21 7.87,47.92 U10.4
  Top 0.406: C5.1 51.41,7.97 51.41,5.86 51.36,5.81 R14.P$2 48.44,2.55 R34.1
  Bottom 0.305: R19.P$2 64.82,35.83 | 64.82,35.83 64.82,37.99 | 64.82,37.99 R20.P$2 | 64.82,37.99 58.5,37.99 D1.C 57.23,39.26 v43.33,39.26 26.49,39.26 25.44,38.21 JP10.2 25.36,37.11 D2.C 26.21,35.17 25.76,34.71 21.72,34.71 21.69,34.74 21.69,37.46 21.01,38.14 v15.98,38.14 13.51,40.58 6.88,40.58 5.92,41.55 U2.4 4.67,42.44 4.32,42.79 4.32,52.06 5.84,53.59 U6.4 | R17.P$1 41.35,62.32 v44.45,62.3 R18.P$1 | 56.49,9.06 v56.49,9.09 56.44,9.09 56.59,4.67 49.94,4.54 49.55,4.49 R14.P$2 | JP24.3 56.69,9.06 | 64.82,35.83 66.73,33.93 U4.1
  Bottom 0.406: JP23.2 36.96,0.91 37.19,0.91 37.26,0.98 48.49,0.98 48.46,2.33 48.44,2.35 R14.P$2
5V  (via drill 0.33)
  Top 0.305: v49.1,17.21 49.15,13.51 U5.39 U5.P$39 | v27.53,17.21 27.48,18.1 27.48,46.42 27.33,46.58 | 27.33,46.58 U1.14 | 27.33,46.58 26.64,47.26 v26.59,47.72 | v61.39,47.64 61.42,55.95 60.71,57.57 D3.C
  Bottom 0.305: v49.1,17.21 v27.53,17.21 | v26.59,47.72 27.2,47.64 v61.39,47.64 | JP9.2 60.45,56.37 D3.C
ANT
  Top 1.016: U1.12 29.44,58.86 29.44,59.28 | R21.P$1 30.1,61.56 29.44,60.9 29.44,59.28 | 29.44,59.28 28.09,60.62 R22.2 26.19,60.62 | R24.1 26.19,60.62 | 26.19,60.62 26.06,60.75 R23.P$1
AUDIO_IN  (via drill 0.33)
  Top 0.305: v31.34,19.04 31.34,13.48 U5.32 U5.P$32 | v45.19,19.09 45.21,19.12 45.21,21.99 46.66,23.44 46.58,25.93 46.56,26.54 46.18,26.71 45.31,27.58 45.21,41.12 44.37,41.95 U1.4 44.37,45.58 v44.37,45.76 | v40.13,63.67 40.03,63.49 40.01,47.59 40.44,46.83 40.46,46.75 40.46,45.81 v40.41,45.69
  Bottom 0.305: v31.34,19.04 31.39,19.09 v45.19,19.09 | J1.24 37.6,66.74 37.64,66.8 37.64,63.67 v40.13,63.67 | v40.41,45.69 40.31,45.79 v44.37,45.76
AUDIO_OUT  (via drill 0.33)
  Top 0.305: v28.98,21.35 28.98,13.66 U5.31 U5.P$31 | v55.24,21.15 55.42,21.33 R27.2 55.98,43.86 R30.P$1 | J1.12 21.65,67.45 21.89,67.45 22.81,66.77 22.84,66.74 32.61,66.74 32.54,66.72 32.54,63.37 32.59,63.34 34.06,63.34 34.14,63.21 v34.14,46.65
  Bottom 0.305: v28.98,21.35 29.06,21.28 51.79,21.35 52.76,20.75 v55.24,21.15 | v34.14,46.65 34.29,46.7 56.77,46.7 57.15,45.97 57.15,44.67 57.96,43.86 R30.P$1
BPF  (via drill 0.33)
  Top 0.305: v26.19,25.55 26.19,31.18 U5.11 U5.P$11 | v54.56,25.47 54.63,61.03 54.61,60.47 R1.P$1 | R2.1 55.27,62.3 55.27,63.24 58.36,63.24 v58.22,67.99 | v51.26,75.41 50.88,77.29 48.51,77.31 | 48.49,77.31 48.51,77.31 | 48.51,77.31 48.18,76.83 48.18,73.35 48.16,73.32 48.13,71.95 46.51,68.63 J1.32
  Top 0.508: R1.P$1 R2.1
  Bottom 0.305: v26.19,25.55 26.39,25.5 47.02,25.5 47.78,26.56 52.25,26.56 53.06,25.47 v54.56,25.47 | v58.22,67.99 58.19,68.04 58.19,74.29 56.06,74.26 52.09,74.29 52.09,74.67 v51.26,75.41
BPSK_CONTROL_A  (via drill 0.33)
  Top 0.305: U2.6 12.52,43.53 12.45,43.53 12.39,43.48 12.39,42.18 12.01,41.8 9.09,41.8 9.09,43.17 9.14,43.22 U10.6 | U5.9 U5.P$9
  Top 0.406: 31.77,33.88 v31.75,44.82
  Top 0.61: U5.9 31.77,33.88
  Bottom 0.305: JP6.1 32.94,44.82 v31.75,44.82
  Bottom 0.406: 31.6,44.98 U2.6
  Bottom 0.61: v31.75,44.82 31.6,44.98
BPSK_CONTROL_B  (via drill 0.33)
  Top 0.305: U6.6 12.32,55.01 12.32,53.33 12.29,53.36 9.63,53.36 9.17,53.82 9.17,54.5 9.07,54.6 U9.6
  Top 0.406: v28.45,54.58 28.45,37.64 28.47,37.64 28.47,33.09 28.75,32.71 U5.P$10 U5.10
  Top 0.61: U5.P$10 28.75,32.09
  Bottom 0.305: v28.45,54.58 28.88,55.01 JP8.1
  Bottom 0.406: v28.45,54.58 27,56.02 14.45,56.02 14.15,56.33 U6.6
BPSK_PWM_A
  Top 0.305: U10.1 11.63,48.81 11.66,48.84 | U5.19 U5.P$19
  Top 0.406: 11.66,48.84 11.66,50.06 11.28,50.44 7.04,50.44 6.6,50.01 U2.1
  Top 0.61: U5.P$19 5.92,38.47 5.92,40.45 5.64,40.53 4.34,40.91 4.42,41.34 4.42,49.45 5.13,50.06 U2.1
BPSK_PWM_B
  Top 0.305: U6.1 5.77,62.88
  Top 0.406: 5.77,62.88 10.97,62.88 11.61,61.28 U9.1 | 4.62,59.45 4.65,51.43
  Top 0.61: U6.1 4.27,60.04 4.27,59.89 4.62,59.45 | 4.65,51.43 3.4,49.62 3.4,49.42 3.35,49.37 U5.P$20 U5.20
GND  (via drill 0.33)
  Top 0.305: J1.9 18.67,63.95 v19.93,63.21 | J1.25 40.13,66.67 42.93,66.82 J1.30 43.94,70.38 43.97,70.4 43.97,71.04 43.56,71.44 J3.5 43.56,72 42.6,72.97 42.6,73.79 J2.GND | v20.5,53.21 20.52,53 U8.7 | v10.24,57.27 10.34,57.17 U9.7 | v10.26,46.09 10.41,45.94 U10.7 | J2.GND2 36.07,73.25 34.85,72.79 33.86,73.27 R4.2 | R2.2 R1.P$2 | D9.C 28.07,78.44 LED2.K | D10.C 51.5,78.58 LED3.K | D11.C 0.89,51.69 LED4.K | LED5.K 1.21,58.55 D12.C | J1.34 48.77,68.28 48.77,69.89 48.74,69.92 48.67,69.92 48.69,69.95 48.77,69.95
  Top 0.406: J1.6 13.41,68 | LED1.K 64.4,79.08 D8.C
  Top 0.508: 13.41,68 13.41,70.53 v14.45,71.66
  Bottom 0.305: U7.7 22.05,53.21 v20.5,53.21 | U6.7 12.04,57.27 v10.24,57.27 | U2.7 12.17,46.09 v10.26,46.09
  Bottom 0.813: 9.84,73.2 v10.62,73.2 | 10.2,75.96 v10.59,75.96
  other vias: 18.62,77.83 16.22,70.64 73.98,21.97 16.99,74.58 22.97,71.85 11.35,17.46 12.09,71.77 67.22,57.35 13.54,74.72 53.16,2 20.76,75.06 21.58,70.83 28,0.97 56.16,42.65 75.04,48.01 64.38,33.8 79.37,32.42 57.28,34.55 66.26,19.64 61.33,42.16 50.8,40.25 6.27,51.87 63.79,27.05 39.81,5.89 12.34,27.95 31.41,73.15 25.4,57.97 26.97,58.66 27.81,57.69 29.16,56.45 30.66,56.7 30.76,57.97 30.76,59.8 24.48,53.45 22.45,63.33 22,58.48 20.27,58.53 18.39,58.6 17.55,59.9 17.4,62.52 14.45,62.9 14.58,59.98 12.22,51.06 14.66,46.16 13.08,62.87 23.05,72.99 23.1,74.77 10.71,71.85 47.05,77.84 19.49,70.73 25.29,70.94 42.23,70.81 44.65,54.06 41.43,54.21 26.34,49.69 17.32,49.18 37.08,45.73 41.3,38.08 50.29,36.94 75.25,40.67 15.96,9.24 72.83,35.13 30.33,49.66 2.36,38.92 60.62,72.71 45.66,73.7 28.96,62.62 24.97,63.35 35.81,57.59 13.94,54.92 16,53.5 71.07,4.92 56.13,3.45 56.86,79.06 61.4,78.94 56.7,69.92 13.38,71.85 13.44,76.04 12.14,76.22 14.2,57.84 14.73,49.49 2.44,40.82 5.43,46.16 2.36,36.61 4.52,39.66 4.52,37.88 4.6,36.28 7.34,39.71 7.24,36 7.21,37.73 0.71,40.57 3.61,55.53 5.28,64.29 48.68,69.89 53.66,69.95 39.13,75.03 39.05,78.25 49.8,28.28 55.38,18.37 59.23,56.29
  pour Bottom: 0,75.23 0,5 arc90 5,0 75.23,0 arc90 80.23,5 80.23,75.23 arc90 75.23,80.23 5,80.23 arc90
  pour Top: 0,75.23 0,5 arc90 5,0 75.23,0 arc90 80.23,5 80.28,75.23 arc90 75.23,80.23 5,80.23 arc90
MIC_IN  (via drill 0.33)
  Top 0.305: U1.8 47.42,58.91 v47.42,56.58 | C9.1 55.96,57.63 C7.2
  Bottom 0.305: v47.42,56.58 47.47,56.63 56.11,56.63 57.1,57.63 C7.2
N$1
  cutout Top: 2.55,77.53 2.58,71.47 9.27,71.44 9.19,77.49
N$2
  cutout Bottom: 2.5,77.62 2.55,71.46 9.31,71.41 9.23,77.56
N$3
  Bottom 0.305: R9.P$2 1.78,48.94 1.78,52.04 2.82,53.08 LED4.A
N$4
  Bottom 0.305: R10.P$2 2.21,61.64 2.21,58.84 2.82,58.23 LED5.A
N$5
  Top 0.305: C9.2 55.91,55.09 C7.1 55.6,53.66 55.58,53.61 R29.P$1 57.28,52.06 55.58,53.54 55.5,52.82 R28.1 55.5,49.57 55.52,49.55 55.7,49.55 | C6.1 57.15,49.55 55.7,49.55 | R30.P$2 55.88,46.4 R27.1 55.47,45.99 C8.2 55.7,48.05 55.7,49.55
N$6
  Top 0.508: LED1.A R11.P$2
N$7  (via drill 1.02)  (7 unrouted)
  other vias: 59.79,15.72 62.33,15.72 64.87,15.72 69.95,15.72 67.41,15.72 72.49,15.72 75.03,15.72 77.57,15.72
N$8  (via drill 0.41)
  Top 0.635: L1.2 9,74.47 v7.99,74.47 X11.ANTENNA
N$9
  Bottom 0.508: LED2.A R12.P$2
N$10
  Top 0.508: L2.1 14.36,73.34 | C1.2 15.73,73.32
  Top 0.762: 14.36,73.34 C1.2 | 15.73,73.32 C2.2
N$11
  Top 0.508: LED3.A R13.P$2
N$12  (via drill 1.02)  (7 unrouted)
  other vias: 59.79,13.18 62.33,13.18 64.87,13.18 69.95,13.18 67.41,13.18 72.49,13.18 75.03,13.18 77.57,13.18
N$14  (via drill 1.02)  (7 unrouted)
  other vias: 59.89,28.39 62.43,28.39 64.97,28.39 70.05,28.39 67.51,28.39 72.59,28.39 75.13,28.39 77.67,28.39
N$15  (via drill 1.02)  (7 unrouted)
  other vias: 59.89,25.85 62.43,25.85 64.97,25.85 70.05,25.85 67.51,25.85 72.59,25.85 75.13,25.85 77.67,25.85
N$16  (via drill 1.02)  (7 unrouted)
  other vias: 59.89,23.31 62.43,23.31 64.97,23.31 70.05,23.31 67.51,23.31 72.59,23.31 75.13,23.31 77.67,23.31
N$17  (via drill 1.02)  (7 unrouted)
  other vias: 59.89,20.77 62.43,20.77 64.97,20.77 70.05,20.77 67.51,20.77 72.59,20.77 75.13,20.77 77.67,20.77
N$18  (via drill 1.02)  (7 unrouted)
  other vias: 59.89,18.23 62.43,18.23 64.97,18.23 70.05,18.23 67.51,18.23 72.59,18.23 75.13,18.23 77.67,18.23
N$19  (via drill 1.02)  (7 unrouted)
  other vias: 59.79,10.64 62.33,10.64 64.87,10.64 69.95,10.64 67.41,10.64 72.49,10.64 75.03,10.64 77.57,10.64
N$20
  Top 0.305: 27.33,70.91 27.3,70.91
N$22  (via drill 0.33)
  Top 0.305: v49.96,44.85 50.11,45 50.11,61.08 50.6,61.56 50.6,63.57 51.59,64.56 J1.35
  Bottom 0.305: JP6.2 33.83,44.85 v49.96,44.85
N$23
  Top 0.305: R4.1 34,76.04 37.67,76.04 37.59,75.97 J2.B5
N$24
  Top 0.305: R3.1 44.72,76.09 40.59,76.09 J2.A5
N$25  (via drill 0.33)
  Top 0.305: v34.82,55.03 35.08,55.29 35.08,66.9 33.98,68 J1.22
  Bottom 0.305: JP8.2 30.91,55.03 v34.82,55.03
N$27
  Top 0.406: D8.A 65.46,77.3 R7.2
N$28
  Top 0.762: L3.1 L4.2
N$29
  Top 0.305: D9.A 28.91,77.27 R8.2
N$30
  Top 0.305: R15.2 51.97,73.49 D10.A
N$31
  Top 0.305: D11.A 2.74,51.41 2.74,44.57 2.42,44.25 R16.2
N$32
  Top 0.305: D12.A 3.25,60.15 R33.2
N$50
  Top 0.635: L1.1 12.51,74.28 L2.2
PB  (via drill 0.33)
  Top 0.305: v18.64,24.53 18.62,31.21 U5.14 U5.P$14 | v73.86,24.48 73.81,24.38 v73.81,70.96 | S1.2 55.4,77.26 v55.4,73.6 61.65,73.6 v62.71,74.59
  Bottom 0.305: J1.37 55.38,66.74 55.38,69.67 55.4,69.68 v55.4,73.6 | v18.64,24.53 46,24.53 46.79,23.39 53.26,23.39 54.08,24.58 73.86,24.53 v73.86,24.48 | v73.81,70.96 72.92,71.85 68.29,71.83 65.53,74.59 v62.71,74.59
PD  (via drill 0.33)
  Top 0.305: U7.6 23.39,52.01 23.39,51.15 22.55,50.31 22.53,50.31 22.53,49.02 22.5,48.99 | 22.5,48.99 19.99,48.99 19.25,49.73 U8.6 | 22.5,43.05 22.5,14.6 U5.29 U5.P$29 | 22.5,43.05 22.5,48.99 | U1.2 37.55,42.99 v36.58,42.99 | v23.44,42.99 23.39,43.05 22.5,43.05 | v65.38,63.37 65.38,63.31 v65.48,43.58
  Bottom 0.305: v23.44,42.99 v36.58,42.99 36.58,41.88 36.65,41.78 59.05,41.72 60.94,43.6 64.16,43.6 v65.48,43.58 | J1.40 60.97,63.34 v65.38,63.37
PI_3V3  (via drill 0.33)
  Top 0.305: U5.12 U5.P$12 D2.A | v31.42,58.84 31.49,46.66 | 31.49,46.66 v31.49,46.55 | v31.49,46.55 31.5,46.04 31.5,45.86 30.89,45.26 30.89,41.12 v30.79,41.01 | v31.49,46.55 31.49,46.66
  Bottom 0.305: D2.A 24.32,36.91 JP10.1 24.56,38.31 24.56,40.23 25.35,41.01 v30.79,41.01 | J1.17 28.88,65.31 28.88,63.59 31.42,62.43 v31.42,58.84 | J1.1 8.43,65.44 8.43,62.38 8.03,61.97 8.03,51.33 10.9,48.46 13.95,48.46 16.46,46.53 v31.49,46.55
PI_5V
  Top 0.305: D6.C 64.34,67.69 D7.C 64.64,65.32 64.64,58.08 62.28,57.47 D3.A
  Top 0.508: J1.2 J1.4
  Bottom 0.305: JP9.1 62.99,56.52 D3.A | J1.4 10.87,67.91 8.2,67.91 7.26,68.85 6.33,68.85 6.15,69.03 1.47,69.03 1.29,69.21 1.29,77.31 1.35,77.31 3.1,79.06 23.39,79.06 25.38,77.08 44.02,77.08 45.11,78.17 45.11,78.2 45.41,78.5 48.01,78.5 49.2,77.31 52.68,77.31 53.39,77.72 55.07,76.88 56.52,76.88 58.32,74.97 61.65,74.14 61.65,69.61 64.34,66.92 D7.C
PI_LED1  (via drill 0.33)
  Top 0.305: v16.05,14.93 U5.26 U5.P$26 | v68.94,14.52 68.78,14.67 68.78,65.98 67.67,67.1 67.67,69.26 v67.72,70.58 | J1.36 51.59,69.69 52.58,70.68 63.72,70.68 R11.P$1
  Top 0.406: R7.1 65.11,70.58 R11.P$1
  Bottom 0.305: v16.05,14.93 16.51,14.95 57.51,14.95 57.94,14.52 v68.94,14.52 | v67.72,70.58 R11.P$1
PI_LED2  (via drill 0.33)
  Top 0.305: 18.75,13.58 v18.75,20.03 | 35.18,20.16 35.18,54.12 36.73,55.67 36.73,63.06 37.64,64.03 37.64,70.17 37.59,70.22 28.65,70.22 27.62,70.25 R12.P$1 | J1.13 22.41,65.86 22.38,66.29 21.51,66.72 19.84,66.74 19.86,66.69 19.86,69.89 19.94,70.05 25.68,70.05 26.53,70.9 R12.P$1 | R8.1 28.42,70.9 R12.P$1 | U5.27 U5.P$27
  Top 0.406: U5.27 18.75,13.58 | v35.13,20.11 35.18,20.16
  Bottom 0.305: 18.82,20.11 v35.13,20.11
  Bottom 0.406: v18.75,20.03 18.82,20.11
PI_RXD  (via drill 0.33)
  Top 0.305: U5.1 51.56,31.26 | 51.56,31.26 v51.56,38.24 | v45.95,38.32 45.82,38.45 45.82,60.55 45.26,61.1 v45.26,70.43 | 51.56,31.26 U5.P$1
  Bottom 0.305: v51.56,38.24 51.49,38.32 v45.95,38.32 | v45.26,70.43 44.98,70.15 32.92,70.15 30.94,72.18 24.89,72.18 23.01,69.82 19.89,69.82 18.57,68.93 J1.10
PI_SCL  (via drill 0.33)
  Top 0.305: v72.25,50.78 72.31,50.72 v72.31,43.4
  Bottom 0.305: J1.5 13.51,65.44 13.51,64.38 8.99,59.48 8.99,59.28 9.02,59.25 9.02,52.7 9.58,52.16 13.23,52.16 14.43,50.95 41.45,51 42.04,50.79 72.24,50.79 v72.25,50.78 | v72.31,43.4 72.25,43.34 JP11.1
PI_SCL3
  Bottom 0.305: J1.18 28.73,67.71 30.58,66.74 32.54,66.72 32.54,63.37 32.51,63.34 34.9,63.34 35.81,62.43 JP4.1 36.11,62.4
PI_SDA  (via drill 0.33)
  Top 0.305: v70.08,48.4 70.05,48.43 v70.08,40.51
  Bottom 0.305: J1.3 10.77,65.28 10.77,63.37 9.17,61.92 8.53,61.28 8.53,52.32 12.42,48.91 14.1,48.96 14.71,48.48 23.72,48.48 25.17,48.43 v70.08,48.4 | v70.08,40.51 69.2,40.59 JP12.1
PI_SDA3
  Bottom 0.305: J1.16 26.51,68 27.91,66.72 29.49,66.69 30,66.14 30,63.95 32.41,62.78 33.38,62.78 33.43,62.73 33.86,62.73 34.19,62.4 34.19,61.21 34.52,60.88 51.94,60.88 51.99,60.83 52.91,61.21 52.91,62.31 JP3.1
PI_TXD  (via drill 0.33)
  Top 0.305: U5.2 48.95,31.34 | 48.95,31.34 v48.95,37.2 | v32.69,37.1 32.64,59.25 31.39,60.47 31.39,63.04 31.45,63.49 v27.46,63.52 | 48.95,31.34 U5.P$2
  Bottom 0.305: v48.95,37.2 48.87,37.13 v32.69,37.1 | v27.46,63.52 27.43,66.34 26.92,66.74 24.87,66.72 17.3,66.72 16.03,67.99 J1.8
PICO_3.3V  (via drill 0.33)
  Top 0.305: D1.A 59.79,36.99 D5.A 58.98,37.2 58.55,36.77 58.55,16.61 v58.19,16.25 | v41.45,16.3 U5.36 U5.P$36
  Bottom 0.305: v58.19,16.25 41.5,16.25 v41.45,16.3
PICO_3.3V1
  Top 0.305: D7.A 66.51,66.33 D6.A
  Bottom 0.305: X1.2 73.84,65.96 D7.A
PICO_RESET  (via drill 0.33)
  Top 0.305: S2.3 S2.4 26,1.91 v26.29,1.9 | v26.29,6.04 26.29,13.35 U5.P$30
  Top 0.406: U5.30 26.29,13.35
  Bottom 0.305: v26.29,6.04 v26.29,1.9
PICO_SCL  (via drill 0.33)
  Top 0.305: U5.7 36.5,31.34 | 36.5,31.34 v36.5,41.04 | R20.P$1 62.76,40.3 | 62.76,40.3 R6.1 | 62.76,40.3 62.74,40.33 v62.74,42.87 | 36.5,31.34 U5.P$7
  Bottom 0.305: v36.5,41.04 36.6,41.14 61.19,41.14 62.28,40.05 R20.P$1 | v62.74,42.87 62.79,42.82 64.92,42.82 66.32,41.42 66.32,38.98 66.34,38.96 66.32,35.58 67.53,34.57 67.61,34.49 71.53,34.49 71.56,34.52 JP1.2
PICO_SCL2
  Top 0.305: U5.5 41.35,31.31 | 41.35,31.31 41.35,35.17 40.79,35.73 40.69,35.73 39.47,36.95 39.47,61.38 38.73,62.12 R17.P$2 | 41.35,31.31 U5.P$5
  Bottom 0.305: 38.58,62.25 R17.P$2 37.1,62.4 JP4.2
PICO_SDA  (via drill 0.33)
  Top 0.305: U5.6 39.01,31.31 | 39.01,31.31 v39.01,35.96 | R19.P$1 62.74,36.29 R5.1 | v67.31,37.59 67.44,37.46 v67.44,32.71 | 39.01,31.31 U5.P$6
  Bottom 0.305: v39.01,35.96 39.22,35.76 R19.P$1 62.2,33.52 63.07,32.66 67.39,32.66 v67.44,32.71 | JP2.2 68.24,37.59 v67.31,37.59
PICO_SDA2  (via drill 0.33)
  Top 0.305: U5.4 44.04,31.26 | 44.04,31.26 v44.07,40.2 | v49.15,40.2 R18.P$2 | 44.04,31.26 U5.P$4
  Bottom 0.305: 49.2,62.38 R18.P$2 51.88,62.32 JP3.2 | v44.07,40.2 v49.15,40.2
PTT  (via drill 0.33)
  Top 0.305: v53.87,7.64 53.85,7.66 53.85,49.85 | 53.85,49.85 53.85,58.72 52.88,59.68 52.88,66.85 54.03,68 J1.38 | U1.3 41.38,43.78 v41.38,49.83 | v52.58,49.83 52.6,49.85 53.85,49.85 | U5.P$22 U5.22
  Bottom 0.305: v53.87,7.64 6.45,7.64 5.84,8.25 5.87,12.9 U5.22 | v41.38,49.83 v52.58,49.83
RF_OUT
  Top 0.406: U8.8 22.53,51.53 22.53,56.48 23.39,57.29 U7.8
  Top 1.016: 23.55,59.91 23.95,59.91 R24.2 23.6,59.56 U7.8 | 23.55,59.91 R26.2 22.33,60.01 22.33,60.88 R25.P$1 | R23.P$2 23.55,61.79 23.55,59.91
RF_PWM
  Top 0.305: J1.7 17.3,67.09 17.31,69.61 | 11.68,44.06 U10.8 | 11.61,55.06 U9.8
  Top 0.406: 17.31,69.61 17.34,71.52 17.79,71.97 | U7.1 16,57.32 21.36,57.32 21.79,56.89 U8.1 | 11.68,44.06 12.34,44.72 12.34,48.81 U2.8 | U6.8 12.32,60.09 12.32,55.77 11.61,55.06
  Top 0.508: 17.79,71.97 C2.1
  Top 0.61: U6.8 15.98,61.41 16.03,61.46 16.03,57.35 U7.1 15.19,57.29 14.78,56.3 14.78,52.37 U2.8
  Top 0.762: C4.2 C3.2 L4.1 17.79,71.97 | C2.1 C1.1
  Top 1.016: U7.1 16.03,57.35 J1.7
RX2  (via drill 0.33)
  Top 0.305: 13.54,31.21 13.54,21.35 17.3,17.52 17.37,8.45 17.37,5.1 v37.95,5.12 | U5.16 U5.P$16
  Top 0.406: U5.16 13.54,31.21
  Bottom 0.406: v37.95,5.12 37.97,5.12 JP23.3
SCL  (via drill 0.33)
  Top 0.305: U4.3 79.6,40.53 79.58,40.58 79.6,40.63 79.6,50.16 79.1,50.82 U3.6 | v75.34,39.01 75.39,38.96 75.39,34.82 76.45,33.75 76.45,7.46 77.55,6.37 77.55,2.91 76.1,1.47 v76.05,1.47
  Bottom 0.305: JP11.2 71.32,40.29 71.32,38.78 71.42,38.88 72.95,38.88 72.61,38.54 JP1.1 | JP1.1 74.31,39.01 74.52,39.01 | U4.3 v75.34,39.01 74.52,39.01 | JP1.1 74.26,38.96 74.47,38.96 74.52,39.01 | v76.05,1.47 75.97,1.39 60.22,1.39 58.65,2.97 JP24.1
SDA  (via drill 0.33)
  Top 0.305: v73.05,42 73.08,41.98 73.08,38.7 72.95,38.83 70.38,38.83 70.36,38.8 v70.36,35.53 70.64,35.53 71.27,34.89 71.27,12.08 71.42,11.93 63.73,11.93 63.68,11.98 63.68,10.2 63.75,10.25 61.11,7.61 61.11,3.91 JP24.2
  Bottom 0.305: U4.4 77.62,42 | 77.62,42 v73.05,42 | v70.36,35.53 70.31,35.58 69.32,35.58 69.33,35.59 JP2.1 69.33,38.99 69.39,39.06 68.2,39.06 68.1,38.96 68.1,40.49 JP12.2 | 77.62,42 76.48,43.15 76.48,52.06 77.78,53.36 U3.5
STM_LED1  (via drill 0.33)
  Top 0.305: v10.85,14.95 10.85,13.56 U5.24 U5.P$24 | R16.1 1.54,42.66 1.04,42.66 0.71,42.99 0.71,45.26 R9.P$1 1.65,46.2
  Bottom 0.305: v10.85,14.95 9.45,16.35 2.03,16.35 1.68,16.71 R9.P$1
STM_LED2  (via drill 0.33)
  Top 0.305: v7.49,41.32 8.97,41.32 9.73,40.68 9.7,17.44 U5.25 U5.P$25 | R33.1 2.68,64.66 R10.P$1
  Bottom 0.305: v7.49,41.32 7.49,63.42 4.65,63.42 3.3,63.44 3.17,63.62 2.13,64.66 R10.P$1
SWTX  (via drill 0.33)
  Top 0.305: v3.5,26.84 3.5,13.58 U5.21 U5.P$21 | v42.8,26.94 42.65,27.1 42.65,57.14 41.71,58.08 41.71,58.41 41.52,58.6 U1.10 41.63,59.02 41.66,60.62 43.99,63.22 J1.29
  Bottom 0.305: v3.5,26.84 3.61,26.94 v42.8,26.94
TEMPERATURE  (via drill 0.33)  (1 unrouted)
  Top 0.305: U5.34 36.42,13.38 | 36.42,13.38 v36.42,9.01 | D4.A 45.9,8.96 R14.P$1 | 36.42,13.38 U5.P$34
  Top 0.406: R34.2 45.9,2.5 R14.P$1
  Bottom 0.305: v36.42,9.01 36.75,8.98 D4.A
TX2
  Top 0.305: 11.1,31.08 11.1,19.65 14.81,15.94 14.88,4.62 15.75,3.75 39.9,3.91 | U5.17 U5.P$17
  Top 0.406: U5.17 11.1,31.08 | 39.9,3.91 40.51,3.29 JP23.4
TXC  (via drill 0.33)
  Top 0.305: 16.23,31.21 v16.23,22.29 | 66.27,22.29 v66.22,60.77 | v53.67,72.97 53.75,72.89 v59.03,72.89 | v59.13,68.68 59.16,68.65 59.16,66.21 61.38,63.99 R32.1 62,61.9 R31.P$1 | U5.15 U5.P$15
  Top 0.406: U5.15 16.23,31.21 | v66.27,22.02 66.27,22.29
  Bottom 0.305: v16.23,22.29 v66.27,22.02 | v66.22,60.77 62,60.75 | J1.26 40.17,66.72 44.63,66.72 45.19,67.28 45.26,67.28 45.26,69.59 45.87,69.97 46.86,69.97 49,72.26 51.38,72.26 52.09,72.97 v53.67,72.97 | v59.03,72.89 59.13,72.79 v59.13,68.68
  Bottom 0.406: 62,60.75 R31.P$1
USB_VBUS  (via drill 0.33)
  Top 0.305: X1.3 75.79,71.82 66.88,71.82 v66.83,71.8 | v62.38,71.8 62.43,71.88 51.28,71.82 | 51.28,71.82 v51.28,74.36 | v46.79,74.82 46.76,71.7 J3.6 | J2.VBUS2 36.91,73.8 36.91,72.89 36.98,72.97 41.81,72.97 41.8,72.98 J2.VBUS1 41.83,73.85 41.81,73.96 41.45,74.77 v41.27,75.38 | 51.28,71.82 R13.P$1 51.4,71.8 R15.1
  Bottom 0.305: v66.83,71.8 v62.38,71.8 | v51.28,74.36 50.72,74.82 50.72,74.9 v46.79,74.82 | v41.27,75.38 42.04,76.09 41.71,76.07 44.65,76.07 44.88,76.09 44.88,73.25 46.1,72.03 J3.6
VBUS
  Top 0.305: U5.40 U5.P$40

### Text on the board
tPlace: Band Pass Filter (BPF) | +X | Antenna | USB-C 5V Input | S1 | Power | Charge | -Y | Transmit | +Y | +Z side | GPIO bus | USB-C breakout | Remove Before Flight | BPF | SR_FRS | U6 | U1 | U7 | U9 | U2 | U8 | MPU6050 IMU 0x68 | U10 | Raspberry Pi Pico | BME280 T/H/P 0x76 | USB | AMSAT(R) CubeSat Simulator Pico v0.1 / (c) CC-BY-NC-SA+ - 2022 AMSAT | KU2Y-KI6ZUM-WD6DRI | CubeSatSim.org | Serial for Camera or GPS | SCL | SDA | 3.3V | GND | -X | GND | 3.3V | RX2 | TX2
bPlace: Mount J1 stacking header or / female header on bottom. | Bridge JP6 and JP8 / if the BPSK analog / switches are on / another board. | -Z side
tNames: +
bNames: If Pi Zero is in use, cut: / JP3, JP4, JP9, JP10, JP11, / JP12 and install D2 and D3.

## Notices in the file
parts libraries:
SparkFun-Aesthetics: Licensing: Creative Commons ShareAlike 4.0 International - https://creativecommons.org/licenses/by-sa/4.0
SparkFun-Connectors: Licensing: CC v3.0 Share-Alike You are welcome to use this library for commercial purposes.
